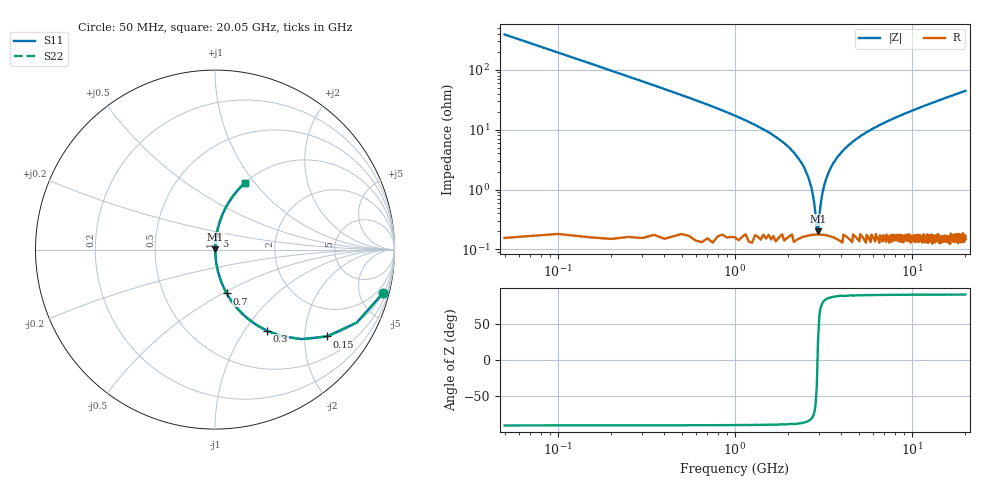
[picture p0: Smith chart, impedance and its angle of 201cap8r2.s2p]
! AVX Thin Film Operation		Date: May 2007
! Description: Accu-P® Series, Thin Film, SMD, RF Capacitor
! Part Number: 0201ZK8R2ABS
! 50 MHz  -  20.05 GHz
! Serial Measurements
# MHZ S MA R 50
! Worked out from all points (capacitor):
!   401 points, 50 MHz to 20.05 GHz, reference 50 ohm
!   read as one part in series: C = 8.2 pF near 150 MHz
!   lowest |Z| = 201 mohm at 2.95 GHz (marker M1)
!   series resonance near 2.929 GHz, so ESL is about 360 pH
!   S11 on the Smith chart (normalised r, x): 50 MHz: 1.01, -7.76; 150 MHz: 1.00, -2.58; 300 MHz: 1.00, -1.28; 700 MHz: 1.00, -0.52; 5 GHz: 1.00, +0.15; 20.05 GHz: 1.00, +0.89
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50  0.968 -14.4  0.25 75.5  0.25 75.5  0.968 -14.4
150  0.79 -37.7  0.612 52.2  0.612 52.2  0.79 -37.7
300  0.539 -57.3  0.841 32.6  0.841 32.6  0.539 -57.3
450  0.388 -67.0  0.92 22.8  0.92 22.8  0.388 -67.0
700  0.253 -75.0  0.966 14.6  0.966 14.6  0.253 -75.0
1900  0.059 -85.1  0.997 3.4  0.997 3.4  0.059 -85.1
2350  0.029 -85.3  0.998 1.7  0.998 1.7  0.029 -85.3
2650  0.013 -82.6  0.998 0.8  0.998 0.8  0.013 -82.6
2750  0.008504 -79.0  0.998 0.5  0.998 0.5  0.008504 -79.0
2850  0.003947 -66.7  0.998 0.2  0.998 0.2  0.003947 -66.7
2950  0.001807 31.0  0.998 -0.1  0.998 -0.1  0.001807 31.0
3000  0.003515 63.7  0.998 -0.2  0.998 -0.2  0.003515 63.7
3100  0.007656 77.9  0.998 -0.4  0.998 -0.4  0.007656 77.9
3200  0.012 81.8  0.998 -0.7  0.998 -0.7  0.012 81.8
3400  0.02 84.4  0.998 -1.1  0.998 -1.1  0.02 84.4
3950  0.04 85.5  0.998 -2.3  0.998 -2.3  0.04 85.5
5000  0.074 84.6  0.996 -4.2  0.996 -4.2  0.074 84.6
6750  0.123 82.2  0.991 -7.1  0.991 -7.1  0.123 82.2
10050  0.203 77.8  0.978 -11.7  0.978 -11.7  0.203 77.8
13400  0.277 73.6  0.959 -16.1  0.959 -16.1  0.277 73.6
16750  0.344 69.6  0.937 -20.1  0.937 -20.1  0.344 69.6
20050  0.405 65.9  0.913 -23.9  0.913 -23.9  0.405 65.9
